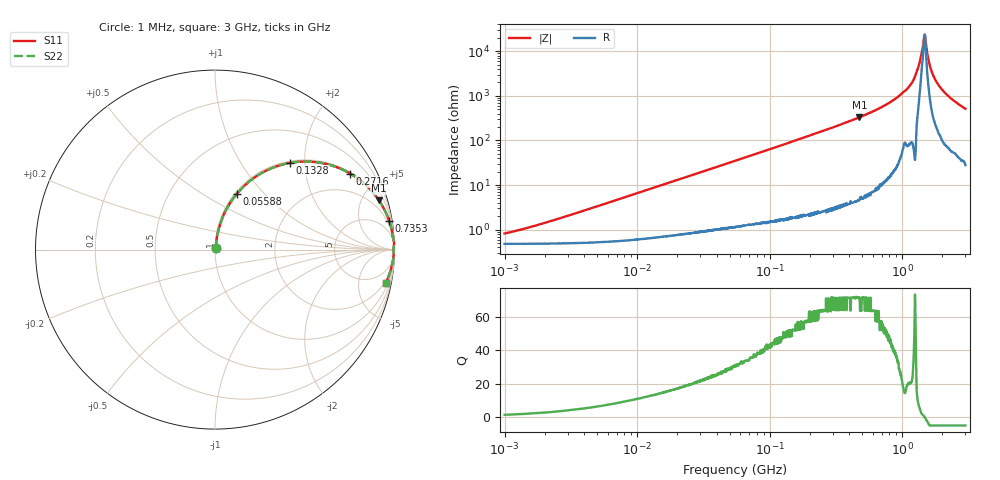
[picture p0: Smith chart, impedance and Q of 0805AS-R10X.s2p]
!s-Parameter Generated by FASTRON Sdn. Bhd.
!FASTRON P/N : 0805AS-R10X
!Keysight Technologies: E4991B_MY54100416_A.01.15
!Date: Mon Jun 15 12:51:56 2026
!Version  :Rev01  Mon Jun 15 12:51:56 2026
!Data & Calibration Information:
!Freq  S11  S21  S12  S22
!PortZ  Port1:50+j0  Port2:50+j0
!When reading reference impedance value at option line is always used.
! Remarks : This data is being provided solely for informational purposes.
# Hz S dB R 50
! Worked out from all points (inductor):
!   1601 points, 1 MHz to 3 GHz, reference 50 ohm
!   read as one part in series: L = 105 nH near 2.216 MHz
!   highest Q = 71.7 at 475.8 MHz (marker M1), where L = 111 nH
!   self-resonance near 1.474 GHz
!   S11 on the Smith chart (normalised r, x): 1 MHz: 1.01, +0.01; 55.88 MHz: 1.02, +0.71; 132.8 MHz: 1.04, +1.69; 271.6 MHz: 1.06, +3.53; 735.3 MHz: 1, +12; 3 GHz: 2, -10
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1000000  -41.80 53.7  -0.04 -0.4  -0.04 -0.4  -41.80 53.7
3804036  -31.90 77.2  -0.05 -1.4  -0.05 -1.4  -31.90 77.2
1.447069e7  -20.60 80.6  -0.10 -5.3  -0.10 -5.3  -20.60 80.6
5.504702e7  -9.68 69.0  -0.59 -19.1  -0.59 -19.1  -9.68 69.0
5.587962e7  -9.57 68.7  -0.61 -19.4  -0.61 -19.4  -9.57 68.7
1.328058e8  -3.89 49.1  -2.43 -39.7  -2.43 -39.7  -3.89 49.1
2.083556e8  -2.00 36.5  -4.52 -52.6  -4.52 -52.6  -2.00 36.5
2.716345e8  -1.27 29.3  -6.20 -59.8  -6.20 -59.8  -1.27 29.3
4.75755e8  -0.41 16.7  -10.80 -72.5  -10.80 -72.5  -0.41 16.7
7.352784e8  -0.14 9.3  -15.80 -79.6  -15.80 -79.6  -0.14 9.3
7.925923e8  -0.12 8.2  -16.90 -80.6  -16.90 -80.6  -0.12 8.2
1.059487e9  -0.07 4.3  -22.50 -81.9  -22.50 -81.9  -0.07 4.3
1.194682e9  -0.03 2.8  -26.30 -84.8  -26.30 -84.8  -0.03 2.8
1.307284e9  -0.02 1.4  -31.90 -83.1  -31.90 -83.1  -0.02 1.4
1.437675e9  -0.04 0.3  -42.70 -49.7  -42.70 -49.7  -0.04 0.3
1.474099e9  -0.04 0.0  -47.30 -5.5  -47.30 -5.5  -0.04 0.0
1.519029e9  -0.04 -0.4  -42.50 56.9  -42.50 56.9  -0.04 -0.4
1.589003e9  -0.03 -0.9  -35.50 75.9  -35.50 75.9  -0.03 -0.9
1.653904e9  -0.04 -1.5  -31.70 80.3  -31.70 80.3  -0.04 -1.5
1.827992e9  -0.05 -2.8  -26.10 81.8  -26.10 81.8  -0.05 -2.8
2.244273e9  -0.10 -5.8  -19.90 80.3  -19.90 80.3  -0.10 -5.8
3e9  -0.25 -10.9  -14.50 76.0  -14.50 76.0  -0.25 -10.9
